FUNCTION_BLOCK FB_LN_IED_LD1_LEDGGIO7 EXTENDS FB_AcsiCommonLogicalNodeClass
VAR_INPUT
	NamPlt: FB_DO_IED_LD1_LEDGGIO7_NamPlt := (sClass:='LPL', bLinkResult:=THIS^.AddDataToContainer(ipData:=NamPlt));
	Beh: FB_DO_IED_LD1_LEDGGIO7_Beh := (sClass:='ENS', bLinkResult:=THIS^.AddDataToContainer(ipData:=Beh));
	Health: FB_DO_IED_LD1_LEDGGIO7_Health := (sClass:='ENS', bLinkResult:=THIS^.AddDataToContainer(ipData:=Health));
	Mod_: FB_DO_IED_LD1_LEDGGIO7_Mod := (sObjectName:='Mod', sClass:='ENC', bLinkResult:=THIS^.AddDataToContainer(ipData:=Mod_));
	AnOut1: FB_DO_IED_LD1_LEDGGIO7_AnOut1 := (sClass:='APC', bLinkResult:=THIS^.AddDataToContainer(ipData:=AnOut1));
	SPCSO1: FB_DO_IED_LD1_LEDGGIO7_SPCSO1 := (sClass:='SPC', bLinkResult:=THIS^.AddDataToContainer(ipData:=SPCSO1));
	DPCSO1: FB_DO_IED_LD1_LEDGGIO7_DPCSO1 := (sClass:='DPC', bLinkResult:=THIS^.AddDataToContainer(ipData:=DPCSO1));
	ISCSO1: FB_DO_IED_LD1_LEDGGIO7_ISCSO1 := (sClass:='INC', bLinkResult:=THIS^.AddDataToContainer(ipData:=ISCSO1));
END_VAR
VAR
END_VAR

END_FUNCTION_BLOCK
